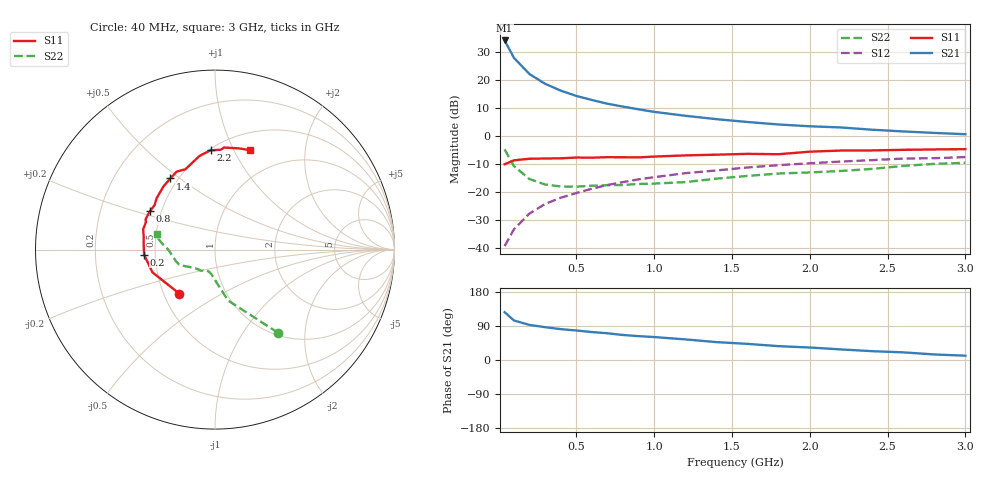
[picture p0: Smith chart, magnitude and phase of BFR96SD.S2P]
! Filename:  BFR96SD.S2P  Version:  2.0
! Philips part #: BFR96S  Date: Jul 1990
! Bias condition: Vce=5V, Ic=70mA
#  MHz  S  MA  R  50
! Freq  S11  S21  S12  S22  !GUM [dB]
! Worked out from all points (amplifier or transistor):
!   21 points, 40 MHz to 3 GHz, reference 50 ohm
!   highest |S21| = 34.1 dB at 40 MHz (marker M1)
!   |S21| within 3 dB of that: start of sweep to 69.06 MHz
!   unconditionally stable (mu >= 1): 181.3 MHz to end of sweep
!   at 300 MHz: K = 1.04, MAG = 20.2 dB, |S12| = -24.2 dB
!   at 1 GHz: K = 1.07, MAG = 10.0 dB, |S12| = -14.6 dB
!   at 3 GHz: K = 1.06, MAG = 2.6 dB, |S12| = -7.5 dB
!   S11 on the Smith chart (normalised r, x): 40 MHz: 0.60, -0.33; 200 MHz: 0.43, -0.03; 800 MHz: 0.43, +0.22; 1.4 GHz: 0.46, +0.46; 2.2 GHz: 0.51, +0.82; 3 GHz: 0.69, +1.16
40  0.316 -128.9  50.53 126.2  0.011 76.3  0.582 -52.8
100  0.371 -160.1  24.77 104.3  0.022 72.2  0.293 -75.6
200  0.396 -175.9  12.74 92.5  0.042 75.0  0.172 -89.5
300  0.4 174.1  8.554 86.6  0.062 75.8  0.138 -98.8
400  0.403 170.1  6.477 81.5  0.08 75.8  0.127 -105.5
500  0.416 164.2  5.205 77.9  0.097 73.9  0.126 -111.3
600  0.414 158.5  4.405 73.7  0.116 72.2  0.131 -115.5
700  0.422 156.2  3.781 70.6  0.135 71.0  0.134 -117.6
800  0.421 149.6  3.355 66.0  0.152 69.4  0.135 -120.5
900  0.418 143.6  3.006 63.0  0.17 67.9  0.141 -123.6
1000  0.433 138.8  2.709 60.6  0.186 66.6  0.143 -128.2
1200  0.454 129.3  2.305 54.4  0.219 62.8  0.152 -137.3
1400  0.468 122.1  2.008 47.2  0.245 59.6  0.175 -146.7
1600  0.484 116.2  1.786 42.6  0.277 57.5  0.196 -152.4
1800  0.477 110.2  1.613 36.5  0.304 52.6  0.216 -157.3
2000  0.529 99.4  1.499 33.0  0.329 49.6  0.226 -162.5
2200  0.554 92.5  1.428 27.9  0.353 46.7  0.24 -171.4
2400  0.557 86.8  1.302 23.3  0.374 45.0  0.261 179.8
2600  0.571 84.9  1.213 20.2  0.399 41.2  0.295 173.6
2800  0.58 76.4  1.142 14.6  0.405 38.2  0.321 169.4
3000  0.587 70.6  1.082 11.4  0.424 36.6  0.335 164.7
